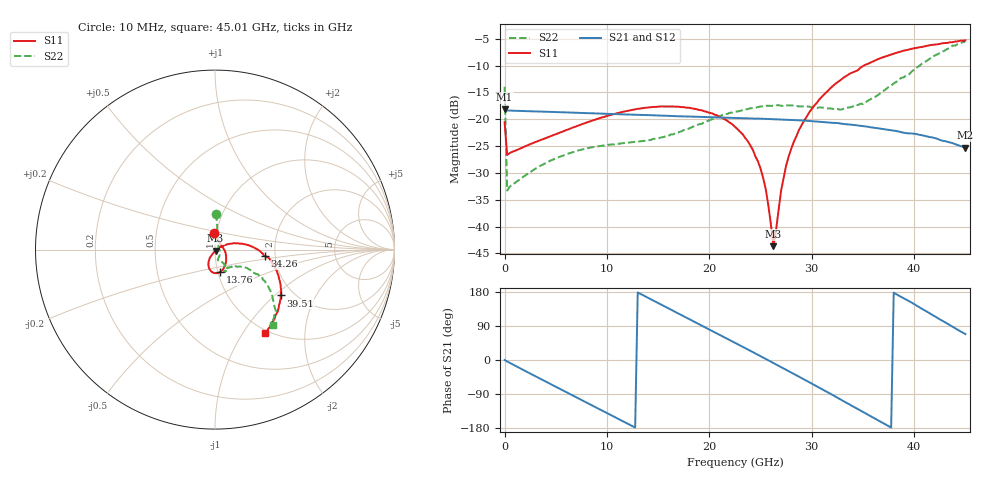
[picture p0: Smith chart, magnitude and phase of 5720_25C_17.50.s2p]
! Device:  ADRF5720
! Description: 0.5dB LSB GaAs MMIC 6-bit Digital Attenuator
! Frequency:  0.000009 -  40 GHz
! Ports:
!	RF1	= Port 1
!	RF2	= Port 2
! Vdd:  3.3 Volt
! Vss:  -3.3 Volt
! Control:  0/3.3 Volt
! State:  17.50 dB attenuation
! Data:  The device was measured using G-S-G Probes on a matrix board.
!  Data was collected using an calibrated 4 port network analyzer.
!  The reference plane for this measurement is at the launchers.
! Note:  Analog Devices supplies this data as a sample of measured data
!  for this product.  Your particular data for this product may vary.
!  Data was taken at 25 degrees C.
!  Analog Devices reserves the right to change this data at anytime.
# GHZ S DB R 45.0
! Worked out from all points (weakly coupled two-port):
!   181 points, 10 MHz to 45.01 GHz, reference 45 ohm
!   highest |S21| = -18.18 dB at 10 MHz (marker M1); lowest = -25.3 dB at 45.01 GHz (marker M2)
!   lowest |S11| = -43.6 dB at 26.26 GHz (marker M3), VSWR 1.01, Z = 45.3 - j0.501 ohm
!   |S11| at or under -10 dB: start of sweep to 35.1 GHz
!   |S22| runs from -33.3 to -5.5 dB; largest |S21 - S12| = 0.00016
!   S11 on the Smith chart (normalised r, x): 10 MHz: 0.97, +0.18; 13.76 GHz: 1.03, -0.26; 34.26 GHz: 1.76, -0.14; 39.51 GHz: 1.72, -1.10; 45.01 GHz: 0.95, -1.26
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0.01  -20.55 94.8  -18.18 -0.1  -18.18 -0.1  -13.96 87.9
0.26  -26.66 10.4  -18.37 -3.9  -18.37 -3.9  -33.28 21.6
3.26  -24.07 -18.7  -18.55 -46.3  -18.55 -46.3  -28.93 -38.5
7.76  -20.78 -47.9  -18.84 -108.9  -18.83 -108.8  -25.53 -70.4
13.76  -17.87 -77.2  -19.22 167.8  -19.22 167.8  -24.00 -71.6
15.26  -17.61 -83.8  -19.30 146.7  -19.30 146.7  -23.41 -67.5
20.26  -18.89 -105.4  -19.62 76.8  -19.63 76.9  -20.00 -58.0
22.76  -21.83 -116.8  -19.78 41.8  -19.78 41.8  -18.55 -59.9
24.01  -24.88 -121.6  -19.86 24.2  -19.86 24.2  -17.96 -61.8
25.01  -29.22 -121.5  -19.89 10.0  -19.90 10.1  -17.61 -63.3
25.51  -33.01 -116.1  -19.93 2.8  -19.93 2.9  -17.50 -64.5
26.26  -43.64 -57.2  -19.98 -8.0  -19.98 -7.9  -17.45 -64.2
27.01  -33.29 18.7  -20.03 -18.8  -20.03 -18.7  -17.48 -65.9
27.76  -26.89 26.1  -20.12 -29.6  -20.12 -29.6  -17.43 -66.2
28.76  -21.99 22.7  -20.21 -44.0  -20.21 -44.0  -17.61 -67.0
30.26  -17.44 15.2  -20.40 -66.2  -20.40 -66.2  -17.77 -65.0
32.26  -13.49 3.9  -20.67 -95.5  -20.67 -95.4  -18.16 -58.0
34.26  -11.08 -7.5  -21.10 -125.7  -21.10 -125.7  -17.30 -45.7
37.76  -7.93 -25.9  -22.04 -178.3  -22.04 -178.3  -13.75 -29.8
39.51  -6.99 -34.8  -22.63 155.4  -22.62 155.5  -11.63 -30.8
42.01  -6.10 -46.5  -23.49 115.0  -23.49 115.1  -8.13 -37.1
45.01  -5.32 -59.3  -25.28 68.3  -25.27 68.4  -5.49 -52.3
